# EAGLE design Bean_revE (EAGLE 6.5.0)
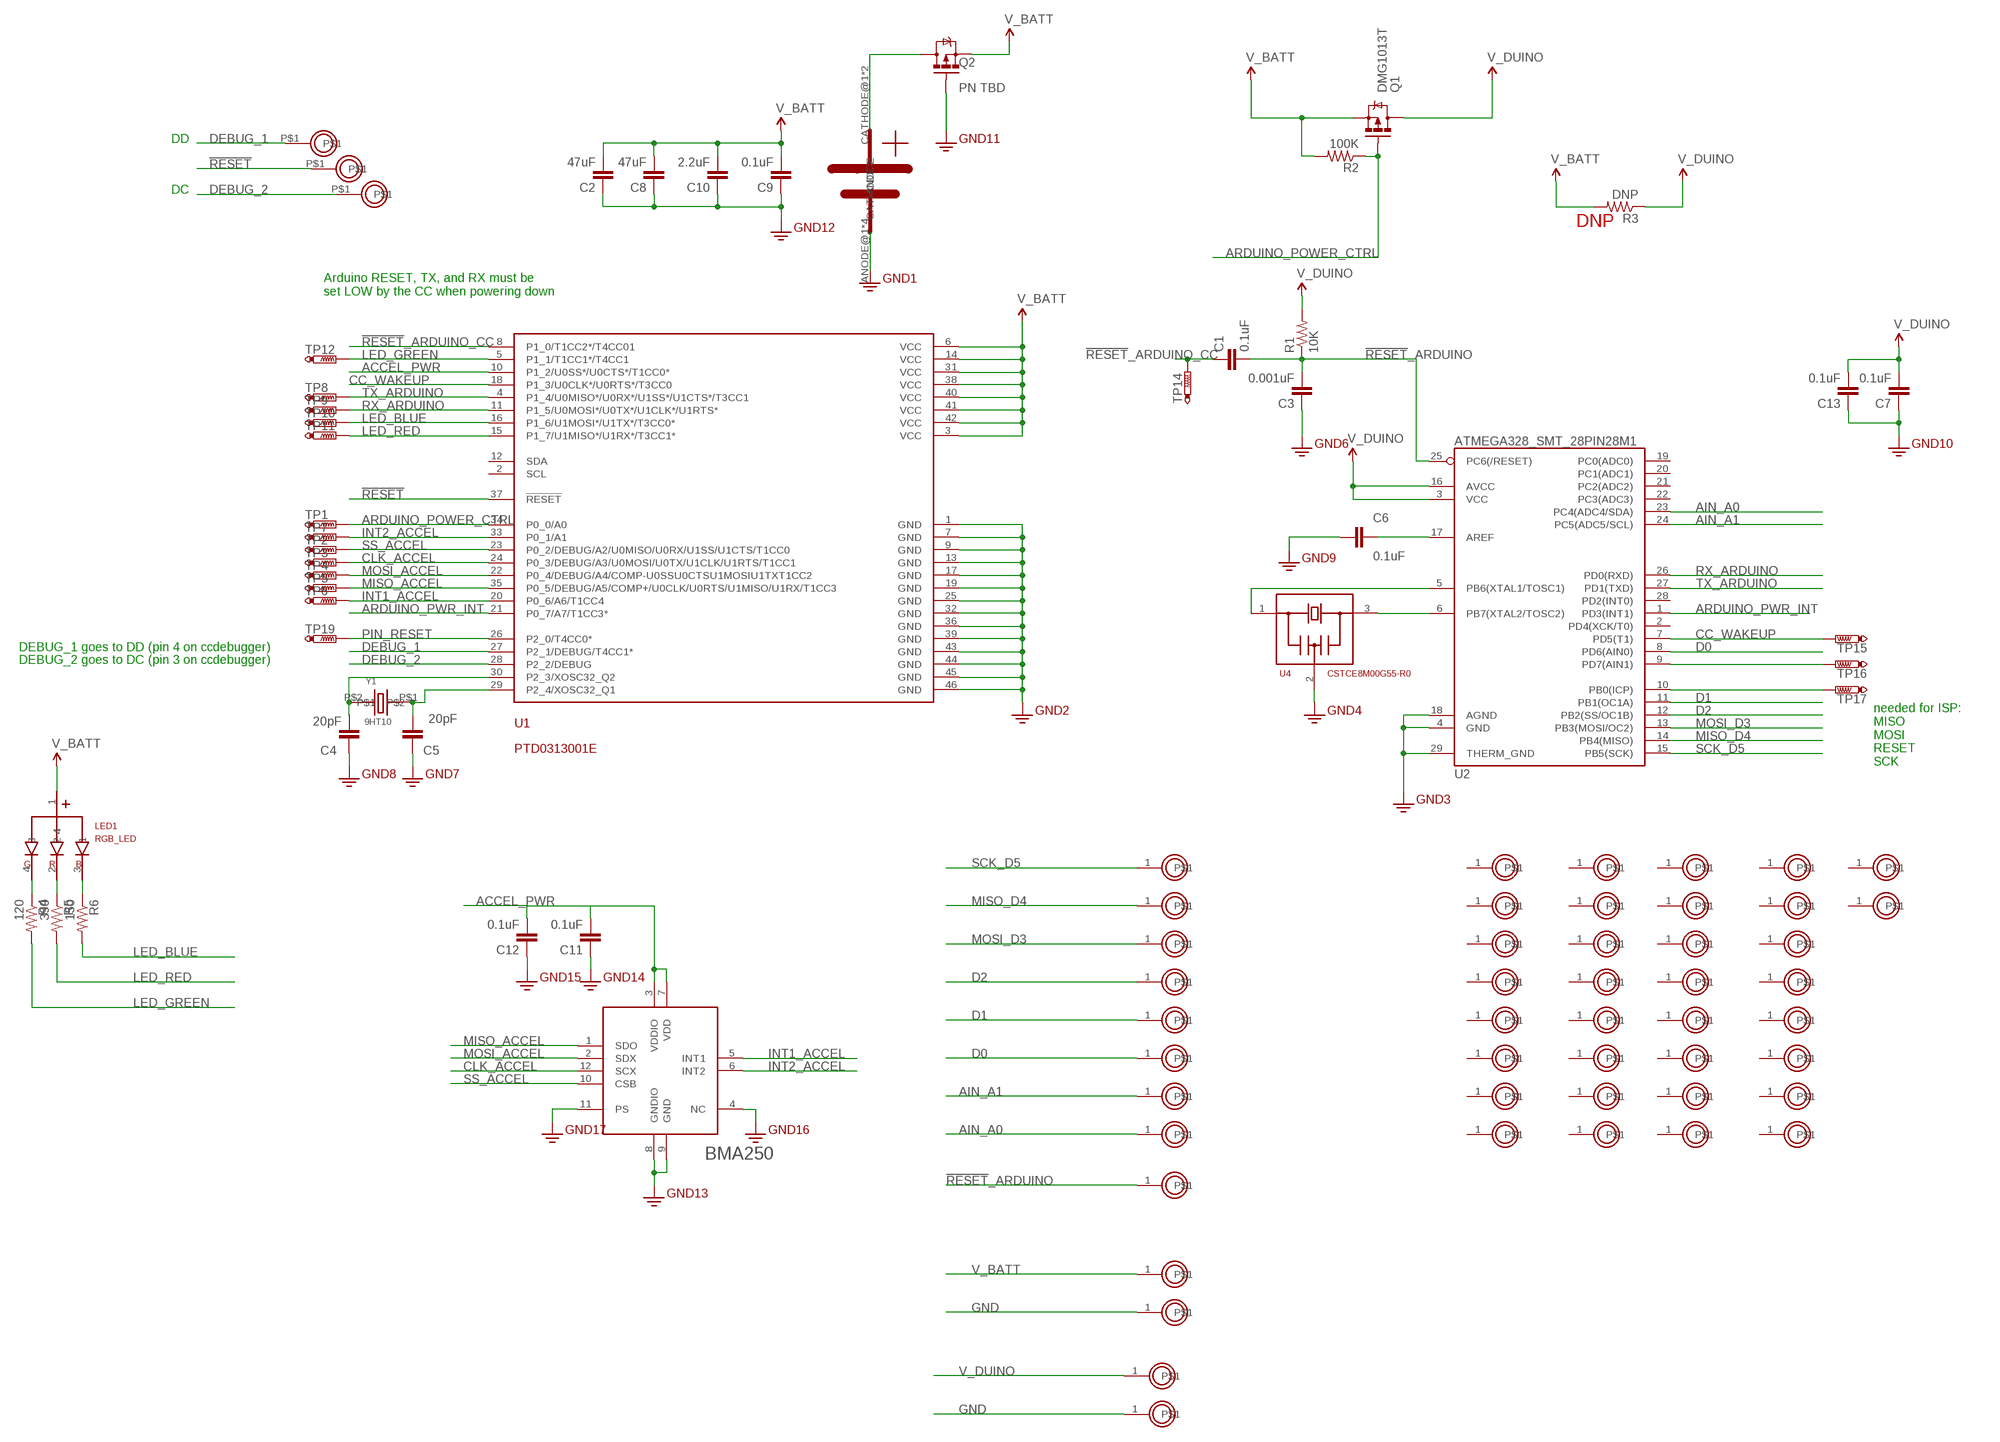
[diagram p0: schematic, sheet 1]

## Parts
C1  0.1uF  CAPACITOR_CERAMIC  [0402]
C2  47uF  CAP0805  [0805]
C3  0.001uF  CAPACITOR_CERAMIC  [0402]
C4  20pF  CAPACITOR_CERAMIC  [0402]
C5  20pF  CAPACITOR_CERAMIC  [0402]
C6  0.1uF  CAPACITOR_CERAMIC  [0402]
C7  0.1uF  CAPACITOR_CERAMIC  [0402]
C8  47uF  CAP0805  [0805]
C9  0.1uF  CAPACITOR_CERAMIC  [0402]
C10  2.2uF  CAP0603-CAP  [0603-CAP]
C11  0.1uF  CAPACITOR_CERAMIC  [0402]
C12  0.1uF  CAPACITOR_CERAMIC  [0402]
C13  0.1uF  CAPACITOR_CERAMIC  [0402]
CN_BATT  CR20324_ELEVATED_PADS  [BK-912-ALT]
LED1  RGB_LED  [SML-LX0404SIUPGUSB]
Q1  DMG1013T  MOSFET-PCHANNEL  [SOT523]
Q2  PN TBD  MOSFET-PCHANNEL  [SOT523]
R1  10K  RESISTOR  [0402]
R2  100K  RESISTOR  [0402]
R3  DNP  RESISTOR  [0402]
R4  120  RESISTOR  [0402]
R5  390  RESISTOR  [0402]
R6  150  RESISTOR  [0402]
TP1  PTR1TP06R  [TP06R]
TP2  PTR1TP06R  [TP06R]
TP3  PTR1TP06R  [TP06R]
TP4  PTR1TP06R  [TP06R]
TP5  PTR1TP06R  [TP06R]
TP6  PTR1TP06R  [TP06R]
TP7  PTR1TP06R  [TP06R]
TP8  PTR1TP06R  [TP06R]
TP9  PTR1TP06R  [TP06R]
TP10  PTR1TP06R  [TP06R]
TP11  PTR1TP06R  [TP06R]
TP12  PTR1TP06R  [TP06R]
TP14  PTR1TP06R  [TP06R]
TP15  PTR1TP06R  [TP06R]
TP16  PTR1TP06R  [TP06R]
TP17  PTR1TP06R  [TP06R]
TP19  PTR1TP14R  [TP14R]
U1  PTD0313001E  [PTD0313001E]
U2  ATMEGA328_SMT_28PIN28M1  [QFN-28-4X4]
U3  BMA250  [BMA250]
U4  CSTCE8M00G55-R0  RESONATOR_3PIN  [CSTCE_G_3PIN_XTAL]
U$1  PROTO_POINT  [1X01]
U$3  PROTO_POINT  [1X01]
U$4  PROTO_POINT  [1X01]
U$5  PROTO_POINT  [1X01]
U$6  PROTO_POINT  [1X01]
U$7  PROTO_POINT  [1X01]
U$8  PROTO_POINT  [1X01]
U$9  PROTO_POINT  [1X01]
U$10  PROTO_POINT  [1X01]
U$11  PROTO_POINT  [1X01]
U$12  PROTO_POINT  [1X01]
U$13  PROTO_POINT  [1X01]
U$14  PROTO_POINT  [1X01]
U$15  PROTO_POINT  [1X01]
U$16  PROTO_POINT  [1X01]
U$17  PROTO_POINT  [1X01]
U$18  PROTO_POINT  [1X01]
U$19  PROTO_POINT  [1X01]
U$20  PROTO_POINT  [1X01]
U$21  PROTO_POINT  [1X01]
U$22  PROTO_POINT  [1X01]
U$23  PROTO_POINT  [1X01]
U$24  PROTO_POINT  [1X01]
U$25  PROTO_POINT  [1X01]
U$26  PROTO_POINT  [1X01]
U$27  PROTO_POINT  [1X01]
U$28  PROTO_POINT  [1X01]
U$29  PROTO_POINT  [1X01]
U$30  PROTO_POINT  [1X01]
U$31  PROTO_POINT  [1X01]
U$32  PROTO_POINT  [1X01]
U$33  PROTO_POINT  [1X01]
U$34  PROTO_POINT  [1X01]
U$35  PROTO_POINT  [1X01]
U$36  PROTO_POINT  [1X01]
U$37  PROTO_POINT  [1X01]
U$38  PROTO_POINT  [1X01]
U$39  PROTO_POINT  [1X01]
U$40  PROTO_POINT  [1X01]
U$41  PROTO_POINT  [1X01]
U$42  PROTO_POINT  [1X01]
U$43  PROTO_POINT  [1X01]
U$44  PROTO_POINT  [1X01]
U$45  PROTO_POINT  [1X01]
U$46  PROTO_POINT  [1X01]
U$49  BEAN_PROGRAM_PIN  [BEAN_PROGAM_PIN]
U$50  BEAN_PROGRAM_PIN  [BEAN_PROGAM_PIN]
U$51  BEAN_PROGRAM_PIN  [BEAN_PROGAM_PIN]
U$52  PROTO_POINT  [1X01]
U$53  PROTO_POINT  [1X01]
Y1  9HT10  [9HT10]

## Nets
!RESET!: U1.37(!RESET!) U$50.P$1
!RESET!_ARDUINO: C1.P$2 C3.P$2 R1.P$1 U2.25(PC6(/RESET)) U$46.1
!RESET!_ARDUINO_CC: C1.P$1 TP14.TP U1.8(P1_0/T1CC2*/T4CC01)
ACCEL_PWR: C11.P$2 C12.P$2 U1.10(P1_2/U0SS*/U0CTS*/T1CC0*) U3.3(VDDIO) U3.7(VDD)
AIN_A0: U2.23(PC4(ADC4/SDA)) U$10.1
AIN_A1: U2.24(PC5(ADC5/SCL)) U$9.1
ARDUINO_POWER_CTRL: Q1.G R2.P$1 TP1.TP U1.34(P0_0/A0)
ARDUINO_PWR_INT: U1.21(P0_7/A7/T1CC3*) U2.1(PD3(INT1))
CC_WAKEUP: TP15.TP U1.18(P1_3/U0CLK*/U0RTS*/T3CC0) U2.7(PD5(T1))
CLK_ACCEL: TP3.TP U1.24(P0_3/DEBUG/A3/U0MOSI/U0TX/U1CLK/U1RTS/T1CC1) U3.12(SCX)
D0: U2.8(PD6(AIN0)) U$8.1
D1: U2.11(PB1(OC1A)) U$7.1
D2: U2.12(PB2(SS/OC1B)) U$6.1
DEBUG_1: U1.27(P2_1/DEBUG/T4CC1*) U$51.P$1
DEBUG_2: U1.28(P2_2/DEBUG) U$49.P$1
GND: C2.1 C3.P$1 C4.P$1 C5.P$1 C6.P$1 C7.P$1 C8.1 C9.P$1 C10.1 C11.P$1 C12.P$1 C13.P$1 CN_BATT.ANODE@1(ANODE) CN_BATT.ANODE@2(ANODE) CN_BATT.ANODE@3(ANODE) CN_BATT.ANODE@4(ANODE) Q2.G U1.1(GND) U1.7(GND) U1.9(GND) U1.13(GND) U1.17(GND) U1.19(GND) U1.25(GND) U1.32(GND) U1.36(GND) U1.39(GND) U1.43(GND) U1.44(GND) U1.45(GND) U1.46(GND) U2.4(GND) U2.18(AGND) U2.29(THERM_GND) U3.4(NC) U3.8(GNDIO) U3.9(GND) U3.11(PS) U4.2 U$45.1 U$53.1 ; supply symbol labelled GND2
INT1_ACCEL: TP6.TP U1.20(P0_6/A6/T1CC4) U3.5(INT1)
INT2_ACCEL: TP7.TP U1.33(P0_1/A1) U3.6(INT2)
LED_BLUE: R6.P$2 TP10.TP U1.16(P1_6/U1MOSI*/U1TX*/T3CC0*)
LED_GREEN: R4.P$2 TP12.TP U1.5(P1_1/T1CC1*/T4CC1)
LED_RED: R5.P$2 TP11.TP U1.15(P1_7/U1MISO*/U1RX*/T3CC1*)
MISO_ACCEL: TP5.TP U1.35(P0_5/DEBUG/A5/COMP+/U0CLK/U0RTS/U1MISO/U1RX/T1CC3) U3.1(SDO)
MISO_D4: U2.14(PB4(MISO)) U$4.1
MOSI_ACCEL: TP4.TP U1.22(P0_4/DEBUG/A4/COMP-U0SSU0CTSU1MOSIU1TXT1CC2) U3.2(SDX)
MOSI_D3: U2.13(PB3(MOSI/OC2)) U$5.1
N$1: U2.5(PB6(XTAL1/TOSC1)) U4.1
N$2: U2.6(PB7(XTAL2/TOSC2)) U4.3
N$3: C4.P$2 U1.30(P2_3/XOSC32_Q2) Y1.P$2
N$4: C5.P$2 U1.29(P2_4/XOSC32_Q1) Y1.P$1
N$6: C6.P$2 U2.17(AREF)
N$23: LED1.4 R4.P$1
N$24: LED1.2 R5.P$1
N$25: LED1.3 R6.P$1
PB0: TP17.TP U2.10(PB0(ICP))
PD7: TP16.TP U2.9(PD7(AIN1))
PIN_RESET: TP19.TP U1.26(P2_0/T4CC0*)
PRE_V_BATT: CN_BATT.CATHODE@1(CATHODE) CN_BATT.CATHODE@2(CATHODE) Q2.D
RX_ARDUINO: TP9.TP U1.11(P1_5/U0MOSI*/U0TX*/U1CLK*/U1RTS*) U2.26(PD0(RXD))
SCK_D5: U2.15(PB5(SCK)) U$3.1
SS_ACCEL: TP2.TP U1.23(P0_2/DEBUG/A2/U0MISO/U0RX/U1SS/U1CTS/T1CC0) U3.10(CSB)
TX_ARDUINO: TP8.TP U1.4(P1_4/U0MISO*/U0RX*/U1SS*/U1CTS*/T3CC1) U2.27(PD1(TXD))
V_BATT: C2.2 C8.2 C9.P$2 C10.2 LED1.1 Q1.S Q2.S R2.P$2 R3.P$2 U1.3(VCC) U1.6(VCC) U1.14(VCC) U1.31(VCC) U1.38(VCC) U1.40(VCC) U1.41(VCC) U1.42(VCC) U$52.1
V_DUINO: C7.P$2 C13.P$2 Q1.D R1.P$2 R3.P$1 U2.3(VCC) U2.16(AVCC) U$1.1
Unconnected: U1.2(SCL) U1.12(SDA) U2.2(PD4(XCK/T0)) U2.19(PC0(ADC0)) U2.20(PC1(ADC1)) U2.21(PC2(ADC2)) U2.22(PC3(ADC3)) U2.28(PD2(INT0)) U$11.1 U$12.1 U$13.1 U$14.1 U$15.1 U$16.1 U$17.1 U$18.1 U$19.1 U$20.1 U$21.1 U$22.1 U$23.1 U$24.1 U$25.1 U$26.1 U$27.1 U$28.1 U$29.1 U$30.1 U$31.1 U$32.1 U$33.1 U$34.1 U$35.1 U$36.1 U$37.1 U$38.1 U$39.1 U$40.1 U$41.1 U$42.1 U$43.1 U$44.1

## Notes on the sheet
- DD
- DC
- DNP
- Arduino RESET, TX, and RX must be
  set LOW by the CC when powering down
- DEBUG_1 goes to DD (pin 4 on ccdebugger)
- DEBUG_2 goes to DC (pin 3 on ccdebugger)
- needed for ISP: 
  MISO
  MOSI
  RESET
  SCK

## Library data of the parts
C1 C3-C7 C9 C11-C13 = BLEduino Bean:CAPACITOR_CERAMIC
C2 C8 = BLEduino Bean:CAP: Capacitor
C10 = SparkFun-Capacitors:CAP: Capacitor
CN_BATT = BLEduino Bean:CR2032
LED1 = BLEduino Bean:RGB_LED
Q1 Q2 = BLEduino Bean:MOSFET-PCHANNEL: Generic PMOSFET
R1-R6 = BLEduino Bean:RESISTOR
TP1-TP12 TP14-TP17 TP19 = testpad:PTR1: TEST PIN
U1 = BLEduino Bean:PTD0313001E
U2 = BLEduino Bean:ATMEGA328_SMT_28PIN
U3 = BLEduino Bean:BMA250: Digital Accelerometer
U4 = BLEduino Bean:RESONATOR_3PIN
U$1 U$3-U$46 U$52 U$53 = BLEduino Bean:PROTO_POINT
U$49-U$51 = BeanLibrary:BEAN_PROGRAM_PIN
Y1 = BLEduino Bean:9HT10

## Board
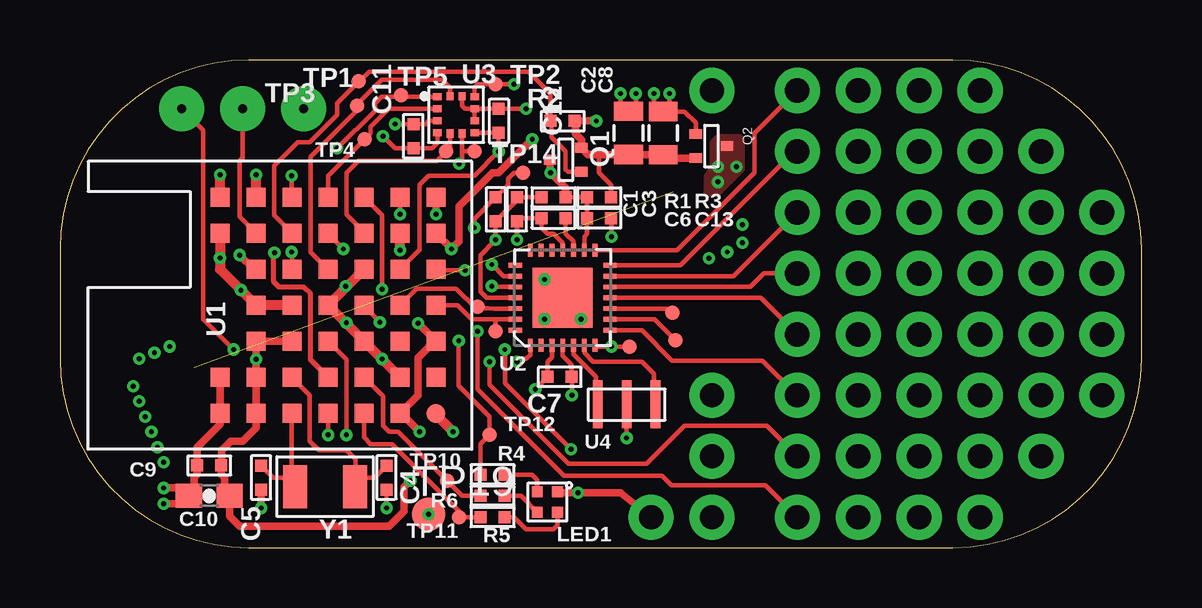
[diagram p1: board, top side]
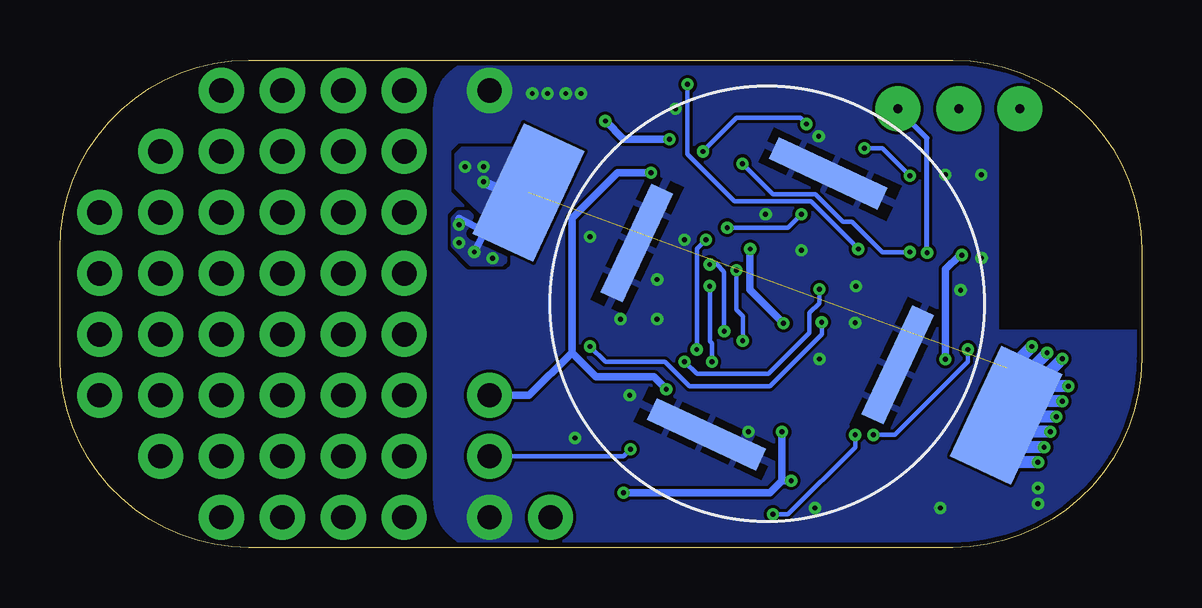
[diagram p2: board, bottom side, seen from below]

Size 45.09 x 20.32 mm. Coordinates in mm from the lower left corner, seen from the top.
Outline: 0,12.45 0,7.87 arc90 7.87,0 37.21,0 arc90 45.09,7.87 45.09,12.45 arc90 37.21,20.32 7.87,20.32 arc90 0,12.45
Copper layers (1*16): Top 0.035mm / dielectric 1.5mm / Bottom 0.035mm
Design rules "default *": minimum track width 7mil, minimum drill 0.15mm, track to track 5mil, track to pad 5mil, pad to pad 5mil, via to via 5mil, smd to smd 1mil, copper to edge 8mil, drill to drill 8mil, minimum pad ring 10mil, minimum via ring 2mil, stop-mask expansion 2mil, vias tented up to drill 13mil, thermal gap 10mil
tRestrict: area 1,10.7 to 5.6,15
bRestrict: area 1,10.7 to 5.6,15; area 8.3,8.7 to 9.4,10.1; area 9.2,9 to 10.3,10.5; area 8.9,7.3 to 10,8.7; area 9.8,7.6 to 10.9,9.1; area 9.5,5.9 to 10.7,7.3; area 10.4,6.2 to 11.5,7.7; area 10.2,4.5 to 11.3,5.9; area 11.1,4.9 to 12.2,6.3; area 19.1,13.9 to 20.2,15.3; area 20,14.2 to 21.1,15.7; area 19.7,12.5 to 20.8,13.9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

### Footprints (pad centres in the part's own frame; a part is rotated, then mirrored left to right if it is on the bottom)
0402 = smd 0.5 x 0.5: P$1 -0.5,0; P$2 0.5,0
0805 = smd 0.8 x 1.2: 1 -0.9,0; 2 0.9,0
0603-CAP = smd 1.1 x 1: 1 -0.85,0; 2 0.85,0
BK-912-ALT = smd 5 x 1: ANODE@1 0,6; ANODE@3 0,-6 | smd 1 x 5: ANODE@2 6,0; ANODE@4 -6,0 | smd 2.79 x 5.08: CATHODE@1 -10.985,0; CATHODE@2 10.985,0
SML-LX0404SIUPGUSB = smd 0.45 x 0.45: 1 0.425,0.425; 2 0.425,-0.425; 3 -0.425,-0.425; 4 -0.425,0.425
SOT523 = smd 0.4 x 0.51: D 0,0.65; G -0.5,-0.65; S 0.5,-0.65
TP06R = smd 0.6 x 0.6: TP 0,0
TP14R = smd 1.4 x 1.4: TP 0,0
PTD0313001E = smd 0.8 x 0.8: 1 1.5,1.5; 2 3,1.5; 3 4.5,1.5; 4 6,1.5; 5 7.5,1.5; 6 9,1.5; 7 10.5,1.5; 8 10.5,3; 9 9,3; 10 7.5,3; 11 6,3; 12 4.5,3; 13 3,3; 14 1.5,3; 15 1.5,4.5; 16 3,4.5; 17 4.5,4.5; 18 6,4.5; 19 7.5,4.5; 20 9,4.5; 21 10.5,4.5; 22 10.5,6; 23 9,6; 24 7.5,6; 25 6,6; 26 4.5,6; 27 3,6; 28 1.5,6; 29 1.5,7.5; 30 3,7.5; 31 4.5,7.5; 32 6,7.5; 33 7.5,7.5; 34 9,7.5; 35 10.5,7.5; 36 10.5,9; 37 9,9; 38 7.5,9; 39 6,9; 40 4.5,9; 41 3,9; 42 1.5,9; 43 1.5,10.5; 44 3,10.5; 45 9,10.5; 46 10.5,10.5
QFN-28-4X4 = smd 0.55 x 0.2: 1 -1.975,1.35; 2 -1.975,0.9; 3 -1.975,0.45; 4 -1.975,0; 5 -1.975,-0.45; 6 -1.975,-0.9; 7 -1.975,-1.35; 15 1.975,-1.35; 16 1.975,-0.9; 17 1.975,-0.45; 18 1.975,0; 19 1.975,0.45; 20 1.975,0.9; 21 1.975,1.35 | smd 0.2 x 0.55: 8 -1.35,-1.975; 9 -0.9,-1.975; 10 -0.45,-1.975; 11 0,-1.975; 12 0.45,-1.975; 13 0.9,-1.975; 14 1.35,-1.975; 22 1.35,1.975; 23 0.9,1.975; 24 0.45,1.975; 25 0,1.975; 26 -0.45,1.975; 27 -0.9,1.975; 28 -1.35,1.975 | smd 2.5 x 2.5: 29 0,0
BMA250 = smd 0.3 x 0.35: 1 -0.75,-0.775; 2 -0.25,-0.775; 3 0.25,-0.775; 4 0.75,-0.775; 7 0.75,0.775; 8 0.25,0.775; 9 -0.25,0.775; 10 -0.75,0.775 | smd 0.35 x 0.3: 5 0.775,-0.25; 6 0.775,0.25; 11 -0.775,0.25; 12 -0.775,-0.25
CSTCE_G_3PIN_XTAL = smd 0.4 x 2: 1 0.07,0; 2 1.27,0; 3 2.47,0
1X01 = drill 1.016 pad 1.88: 1 0,0
BEAN_PROGAM_PIN = drill 0.381 pad 1.88: P$1 0,0
9HT10 = smd 1 x 1.8: P$1 -1.25,0; P$2 1.25,0

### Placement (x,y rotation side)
C1  18.16,14.1 270 top
C2  23.7,17.28 270 top
C3  19.05,14.1 90 top
C4  13.61,2.92 90 top
C5  8.38,2.92 90 top
C6  20.57,13.72 0 top
C7  20.83,7.11 180 top
C8  25.15,17.27 270 top
C9  6.22,3.43 0 top
C10  6.22,2.16 0 top
C11  14.73,17.14 90 top
C12  18.29,17.78 270 top
C13  22.48,13.72 180 top
CN_BATT  15.6,10.16 335 bottom
LED1  20.32,1.91 0 top
Q1  21.08,16.16 90 top
Q2  27.15,16.73 270 top
R1  20.57,14.61 0 top
R2  20.95,17.78 0 top
R3  22.48,14.61 0 top
R4  18.03,3.05 180 top
R5  18.03,1.27 180 top
R6  18.03,2.16 180 top
TP1  12.45,19.43 0 top
TP2  18.16,19.3 0 top
TP3  12.38,18.41 0 top
TP4  12.7,17.02 0 top
TP5  14.22,18.85 0 top
TP6  16.1,16.51 0 top
TP7  17.27,16.51 0 top
TP8  18.16,9.02 0 top
TP9  17.4,10.03 0 top
TP10  16.13,2.79 0 top
TP11  16.64,1.27 0 top
TP12  17.91,4.7 0 top
TP14  19.3,15.62 0 top
TP15  23.75,8.38 0 top
TP16  25.65,8.64 0 top
TP17  25.53,9.78 0 top
TP19  15.37,1.4 0 top
U1  17.18,4.1 90 top
U2  20.95,10.41 90 top
U3  16.51,18.03 270 top
U4  22.35,5.97 0 top
U$1  27.18,6.35 0 top
U$3  30.73,19.05 0 top
U$4  30.73,16.51 0 top
U$5  30.73,13.97 0 top
U$6  30.73,11.43 0 top
U$7  30.73,8.89 0 top
U$8  30.73,6.35 0 top
U$9  30.73,3.81 0 top
U$10  30.73,1.27 0 top
U$11  33.27,19.05 0 top
U$12  35.81,19.05 0 top
U$13  33.27,11.43 0 top
U$14  33.27,16.51 0 top
U$15  35.81,16.51 0 top
U$16  35.81,11.43 0 top
U$17  33.27,13.97 0 top
U$18  35.81,13.97 0 top
U$19  33.27,1.27 90 top
U$20  33.27,3.81 90 top
U$21  33.27,6.35 90 top
U$22  33.27,8.89 90 top
U$23  38.35,13.97 0 top
U$24  35.81,1.27 90 top
U$25  35.81,3.81 90 top
U$26  35.81,6.35 90 top
U$27  35.81,8.89 90 top
U$28  38.35,16.51 0 top
U$29  38.35,11.43 90 top
U$30  38.35,3.81 90 top
U$31  38.35,6.35 90 top
U$32  38.35,8.89 90 top
U$33  40.89,16.51 0 top
U$34  40.89,13.97 0 top
U$35  40.89,6.35 0 top
U$36  40.89,11.43 0 top
U$37  40.89,3.81 0 top
U$38  40.89,8.89 0 top
U$39  38.35,19.05 0 top
U$40  43.43,13.97 0 top
U$41  38.35,1.27 0 top
U$42  43.43,11.43 0 top
U$43  43.43,8.89 0 top
U$44  43.43,6.35 0 top
U$45  27.18,19.05 0 top
U$46  27.18,3.81 0 top
U$49  5.08,18.29 0 top
U$50  7.62,18.29 0 top
U$51  10.16,18.29 0 top
U$52  24.64,1.27 0 top
U$53  27.18,1.27 0 top
Y1  11.05,2.54 0 top

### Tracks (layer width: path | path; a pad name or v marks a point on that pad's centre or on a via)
!RESET!
  Top 0.178: U1.37 7.49,13.78 7.49,16.13 7.62,16.26 U$50.P$1
  Top 0.203: U1.37 8.11,13.1
!RESET!_ARDUINO  (via drill 0.2 pad 0.51)
  Top 0.178: R1.P$1 19.18,14.61 C3.P$2 19.05,14.49 C1.P$2 v18.16,12.83 17.53,12.19 17.53,10.67 17.78,10.41 U2.25 | v18.54,8.27 v18.54,8.26 18.54,6.86 v21.3,4.1
  Bottom 0.178: v18.54,8.26 18.54,12.45 v18.16,12.83 | v21.3,4.1 21.59,3.81 U$46.1
!RESET!_ARDUINO_CC  (via drill 0.2 pad 0.51)
  Top 0.178: v17.27,13.34 17.27,13.71 C1.P$1 18.67,15.11 18.67,15.37 18.92,15.62 TP14.TP | U1.8 v14.18,13.9 v14.17,13.89
  Bottom 0.178: v17.27,13.34 14.73,13.34 v14.17,13.89
ACCEL_PWR  (via drill 0.2 pad 0.51)
  Top 0.178: U3.7 C12.P$2 v18.29,16.51 17.27,15.49 15.37,15.49 14.99,15.11 14.99,12.41 U1.10 | U3.3 15.37,17.78 15.23,17.64 C11.P$2 14.72,17.65 v13.97,17.65
  Bottom 0.178: v18.29,16.51 16.89,17.91 14.22,17.91 v13.97,17.65
AIN_A0  (via drill 0.2 pad 0.51)
  Top 0.178: v18,11.8 18.49,11.31 U2.23 | U$10.1 29.4,2.6 25.49,2.6 25.09,3 21,3 17.4,6.6 v17.4,9.02
  Bottom 0.178: v18,11.8 17.7,11.8 17.4,11.5 v17.4,9.02
AIN_A1  (via drill 0.2 pad 0.51)
  Top 0.178: v18,10.9 18.04,10.86 U2.24 | U$9.1 29.46,5.08 26.04,5.08 24.45,3.5 21.2,3.5 17.91,6.79 v17.91,7.75
  Bottom 0.178: v18,10.9 18,8.6 17.91,8.51 v17.91,7.75
ARDUINO_POWER_CTRL
  Top 0.178: U1.34 8.93,13.85 8.93,15.91 9.91,16.89 10.41,16.89 11.56,18.03 11.56,18.52 12.39,19.36 | 12.39,19.36 12.88,19.84 19.53,19.84 20.45,18.92 R2.P$1 20.5,17.74 20.5,17.09 21.08,16.51 21.08,15.75 21.17,15.66 Q1.G | TP1.TP 12.45,19.36 12.39,19.36
ARDUINO_PWR_INT  (via drill 0.2 pad 0.51)
  Top 0.178: v13.43,10.77 13.43,13.85 U1.21 | v19.05,7.75 19.18,7.87 19.43,7.87 19.61,8.05 U2.1
  Bottom 0.178: v19.05,7.75 18.54,7.24 15.56,7.24 13.84,8.96 13.84,9.78 13.43,10.19 v13.43,10.77
CC_WAKEUP  (via drill 0.2 pad 0.51)
  Top 0.178: U1.18 12.68,10.06 v13.34,9.4 | U2.7 22.36,8.38 v22.99,8.38 TP15.TP
  Bottom 0.178: v13.34,9.4 13.34,8.89 15.49,6.73 18.85,6.73 19.86,7.75 22.35,7.75 v22.99,8.38
CLK_ACCEL
  Top 0.178: 10.96,11.6 U1.24 11.16,11.6 10.44,12.32 10.44,16.28 12.38,18.22 TP3.TP 12.38,18.48 13.41,19.51 15.93,19.51 16.26,19.17 U3.12
D0
  Top 0.178: U$8.1 29.29,7.8 25.52,7.8 24.25,9.06 U2.8
D1
  Top 0.178: U$7.1 29.21,10.41 U2.11
D2
  Top 0.178: U$6.1 29.34,11.43 28.77,10.86 U2.12
DEBUG_1  (via drill 0.2 pad 0.51)
  Top 0.203: U1.27 10.44,7.84 10.44,10.59 10.17,10.86 9.13,10.86 8.91,11.07 8.91,12.27 v8.94,12.29
  Bottom 0.203: v8.94,12.29 8.94,17.07 U$51.P$1
DEBUG_2  (via drill 0.2 pad 0.51)
  Top 0.178: U1.28 v11.18,4.7 | U$49.P$1 5.97,17.4 5.97,9.53 v7.24,8.26
  Bottom 0.178: v11.18,4.7 10.29,4.7 7.24,7.75 v7.24,8.26
GND  (via drill 0.2 pad 0.51)
  Top 0.178: U2.4 20.95,8 21.33,7.63 C7.P$1 v21.34,6.35 | U3.4 15.73,16.88 15.5,16.64 C11.P$1 | U3.9 C12.P$1 v19.43,18.29 | U3.9 U3.8 | U3.9 16.89,18.29 16.76,18.42 U3.11 | v19.05,12.83 C3.P$1 19.17,13.72 C6.P$1 20.07,13.33 20.32,13.08 20.57,13.08 20.95,12.7 U2.18 | U4.2 v23.62,4.57 | Q2.G 26.5,17.7 26.04,18.16 C8.1 | v23.37,18.92 23.37,18.51 C2.1 24,18.48 v24,18.92 | v24.77,18.92 24.77,18.54 25.14,18.17 C8.1 | v25.4,18.92 25.4,18.43 C8.1 | v22.99,12.95 22.99,13.71 C13.P$1 | v20.19,11.18 20.19,10.41 U2.29 | C11.P$1 | C11.P$1 13.96,16.64 v13.46,17.14 | C4.P$1 v13.61,1.65
  Top 0.305: U1.19 12.62,11.6 v11.91,10.89 | U1.44 U1.43 6.68,5.15 5.71,4.19 C9.P$1 5.72,3.06 5.59,2.92 5.59,2.37 | 5.59,2.37 C10.1 | C10.1 5.33,2.16 | 5.59,2.37 5.12,2.37 5.08,2.41 | v4.32,2.49 5.04,2.49 C10.1 | v4.32,1.83 5.04,1.83 C10.1 | C5.P$1 v8.38,1.65 | v15.67,13.89 U1.7
  Top 0.406: U1.19 U1.25 U1.17 U1.13 | U1.32 U1.39 6.68,11.6 v6.68,12.07 | v16.38,4.83 15.68,5.53 U1.1 | U1.45 v6.68,12.07 | v6.68,12.07 v6.67,12.07 | U1.36 v8.18,15.54 | v14.17,12.39 U1.9 | U1.46 v6.68,15.54
  Bottom 0.305: v8.38,1.65 8.51,1.65
  other vias: 11.94,9.37 13.43,7.86 7.54,10.73 20.19,9.53 21.72,9.53
  pour Bottom (rank 3, no thermals): 7.87,20.32 27.43,20.32 arc-90 29.46,18.29 29.46,2.03 arc-90 27.43,0 7.87,0 arc-93 0,8.26 0,12.57 arc-91
INT1_ACCEL
  Top 0.178: U1.20 12.68,13.13 11.94,13.87 11.94,15.62 12.45,16.13 15.72,16.13 TP6.TP 16.26,16.51 16.26,16.66 U3.5
INT2_ACCEL  (via drill 0.2 pad 0.51)
  Top 0.178: v16.64,16 16.76,16.12 16.76,16.51 | 16.76,16.51 U3.6 | U1.33 9.68,12.29 v9.65,12.32 | TP7.TP 16.76,16.51
  Bottom 0.178: v16.64,16 15.37,14.73 13.59,14.73 12.45,13.59 12.06,13.59 10.79,12.32 v9.65,12.32
LED_BLUE
  Top 0.178: U1.16 13.46,6.31 13.46,5.08 13.72,4.83 14.1,4.83 TP10.TP 16.76,2.16 R6.P$2
LED_GREEN  (via drill 0.2 pad 0.51)
  Top 0.178: U1.5 15.72,11.56 v16.89,11.56 | v16.62,8.62 16.62,6.74 17.91,5.46 TP12.TP 17.53,4.33 R4.P$2
  Bottom 0.178: v16.89,11.56 16.89,9.91 16.62,9.64 v16.62,8.62
LED_RED
  Top 0.178: 16.89,1.27 R5.P$2 TP11.TP 16.64,1.52 13.84,4.32 12.95,4.32 12.68,4.6 U1.15
MISO_ACCEL  (via drill 0.2 pad 0.51)
  Top 0.178: 9.68,14.82 U1.35 9.65,14.62 v9.65,15.49 | U3.1 14.29,18.78 | TP5.TP 14.29,18.78 | 14.29,18.78 13.4,18.78 13.13,18.52 13.13,18.21 v11.56,16.64
  Bottom 0.178: v9.65,15.49 10.79,16.64 v11.56,16.64
MISO_D4
  Top 0.178: U$4.1 30.61,16.51 25.86,11.76 U2.14
MOSI_ACCEL
  Top 0.178: U3.2 13.7,18.28 12.95,17.54 12.95,17.27 TP4.TP 11.18,15.49 U1.22
MOSI_D3
  Top 0.178: U$5.1 28.08,11.31 U2.13
N$1
  Top 0.178: U2.5 21.41,8.06 22.35,7.11 22.35,6.86 22.35,6.73 22.35,6.04 U4.1
N$2
  Top 0.178: U2.6 21.86,8.12 22.23,7.75 24.26,7.75 24.77,7.24 24.77,6.03 U4.3
N$3
  Top 0.178: 9.93,7.07 9.93,6.83 10.41,6.35 10.41,4.45 10.79,4.06 11.94,4.06 12.32,3.68 12.32,2.56 Y1.P$2 | Y1.P$2 12.3,2.65 12.32,2.67 | C4.P$2 13.11,2.92 12.3,2.92 Y1.P$2
  Top 0.254: U1.30 9.93,7.07
N$4
  Top 0.178: U1.29 9.65,5.58 9.65,3.05 9.8,2.9 Y1.P$1 | Y1.P$1 9.8,2.56 9.91,2.67 | C5.P$2 8.88,2.92 9.8,2.92 Y1.P$1
N$6
  Top 0.178: U2.17 21.41,12.76 21.08,13.08 21.08,13.71 C6.P$2
N$23
  Top 0.178: R4.P$1 19.68,3.05 19.89,2.84 LED1.4
N$24
  Top 0.178: R5.P$1 18.92,1.27 19.43,0.76 20.57,0.76 20.75,0.93 LED1.2
N$25
  Top 0.178: R6.P$1 19.22,2.16 LED1.3
PB0
  Top 0.178: U2.10 25.34,9.96 TP17.TP
PD7
  Top 0.178: U2.9 24.78,9.51 TP16.TP
PIN_RESET  (via drill 0.2 pad 0.51)
  Top 0.178: U1.26 11.94,7.84 v11.94,4.7 | 14.99,1.4 TP19.TP
  Bottom 0.178: v11.94,4.7 11.94,4.19 14.73,1.4 TP19.TP
  other vias: 15.37,1.4
PRE_V_BATT  (via drill 0.2 pad 0.51)  (1 unrouted)
  Bottom 0.305: CN_BATT.CATHODE@1 27.43,13.08 v27.81,12.32 27.3,13.34 27.43,13.21 28.45,13.72
  Bottom 0.406: 4.32,6.6 4.57,6.6 | 4.57,6.6 4.57,6.1 4.57,5.46 | 5.08,4.83 4.7,4.83 4.7,5.46 | 5.08,4.83 5.64,4.83 CN_BATT.CATHODE@2 | 5.08,4.83 5.08,4.32 | 5.08,4.19 5.21,4.19 5.21,3.56 | 5.59,7.49 5.08,7.49 5.08,6.99 5.08,6.6 4.57,6.6 | v27.43,15.24 26.29,14.73 | 26.29,14.73 arc-59 CN_BATT.CATHODE@1 | 26.29,14.73 arc62 26.16,13.59 26.23,13.45 arc-173 27.05,13.84
  Bottom 0.508: v3.05,6.73 4.32,6.73 | 4.32,6.73 4.32,6.6 | v3.3,6.1 4.57,6.1 | v3.56,5.46 4.57,5.46 4.7,5.46 | v3.81,4.83 5.08,4.83 | v4.06,4.19 5.08,4.19 5.08,4.32 | v4.32,3.56 5.21,3.56 5.33,3.56 5.33,3.43 | v3.3,7.87 4.32,6.86 4.32,6.73 | v3.94,8.13 5.08,6.99 5.21,6.86 | v4.57,8.38 5.46,7.49 5.59,7.49
  other vias: 27.43,15.88 28.19,15.88 28.45,12.7 27.05,12.06 28.45,13.46
  pour Top (no thermals): 28.32,17.14 27.43,17.14 27.18,16.89 27.18,15.88 26.92,15.49 26.92,14.73 27.43,14.73 28.45,15.75 28.45,17.02
  pour Bottom (no thermals): 26.42,15.37 26.67,14.61 26.8,14.35
  pour Bottom: 26.67,11.81 27.94,11.81 28.7,12.57 28.7,13.72 28.45,13.97 28.07,13.97 26.54,12.45 26.54,11.94
  pour Bottom (no thermals): 26.04,16.64 28.32,16.64 28.57,16.38 28.57,14.99 27.94,14.35 27.56,13.97 26.16,13.97 26.04,14.1
RX_ARDUINO
  Top 0.178: U2.26 18.09,9.96 17.84,9.97 17.4,9.97 | 17.4,9.97 17.34,9.97 16.51,10.79 14.87,10.79 U1.11 | TP9.TP 17.4,9.97
SCK_D5
  Top 0.178: U$3.1 28.96,17.27 28.96,15.62 25.72,12.39 U2.15
SS_ACCEL  (via drill 0.2 pad 0.51)
  Top 0.178: 11.18,13.07 U1.23 11.81,12.46 v11.81,12.45 | U3.10 17.29,19.19 17.4,19.3 TP2.TP v18.92,19.3
  Bottom 0.178: v11.81,12.45 13.79,14.43 16.97,14.43 18.92,16.38 v18.92,19.3
TX_ARDUINO
  Top 0.178: U2.27 18.16,9.51 | 18.16,9.51 17.16,9.51 16.57,10.1 U1.4 | TP8.TP 18.16,9.51
V_BATT  (via drill 0.2 pad 0.51)
  Top 0.178: 20.79,2.29 LED1.1 | R3.P$2 22.98,15.12 22.48,15.62 22.48,16.38
  Top 0.305: v14.92,9.35 U1.3 15.61,8.6 14.92,7.91 14.92,6.35 U1.14 14.21,5.6 v14.99,4.83 | Q2.S 25.29,16.23 C8.2 C2.2 22.48,16.38 22.01,16.38 Q1.S 21.73,17 21.5,17.24 21.5,17.74 R2.P$2 v22.35,17.78 | U1.31 U1.40 v8.18,7.85 U1.41 U1.42 8.18,5 7.62,4.45 7.11,4.45 6.73,4.06 C9.P$2 6.72,3.06 6.86,2.92 6.86,2.37 C10.2 7.07,1.31 7.49,0.89 13.72,0.89 14.35,1.52 14.35,2.54 v14.61,2.79 | v7.49,12.19 8.09,11.6 U1.38 | 20.79,2.29 v21.59,2.29 23.37,2.29 U$52.1 | v19.68,17.02 18.29,15.62 18.03,15.62 16.64,14.22 16.64,12.77 v16.32,12.45 15.68,13.09
  Top 0.406: 15.68,13.09 U1.6
  Bottom 0.305: v14.61,2.79 14.99,2.79 | 14.99,2.79 v14.99,4.83 | v8.18,7.85 U1.38 7.58,12.19 v7.49,12.19 | v19.68,17.02 21.59,17.02 v22.35,17.78 | v21.59,2.29 15.49,2.29 14.99,2.79 | v14.92,9.35 16.32,10.75 v16.32,12.45
V_DUINO  (via drill 0.2 pad 0.51)
  Top 0.178: U2.16 21.86,12.96 21.97,13.08 21.97,13.71 C13.P$2 R3.P$1 R1.P$2 | U2.3 20.5,7.93 20.32,7.75 C7.P$2 | C7.P$2 | C7.P$2 20.31,7.11 20.07,6.86 v19.81,6.6 | 20.43,15.64 20.43,15.62 v20.45,15.62
  Top 0.305: R1.P$2 21.07,14.99 v20.45,15.62 20.43,15.64 Q1.D
  Bottom 0.305: 23.75,8.13 23.75,13.72 21.84,15.62 v20.45,15.62 | U$1.1 25.53,6.35 23.75,8.13 | 23.75,8.13 22.73,7.11 C7.P$2 v19.81,6.6

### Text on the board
Document: Bean Revision E | ray@ | P/N: PTD1013012E | punchthrough.com | ck@ | Rev E | Top Silk: tPlace tArt | Bottom Silk: bArt | Layers: 2 | Rectangular Dimensions: 1.775" x 0.8" (45.09mm x 20.32mm) | Finished Thickness: 0.062" | Finish: ENIG | Material: FR4 | Copper Weight: 1oz | Soldermask: Top and bottom | Silkscreen: Top and Bottom | Silkscreen Color: Black | Soldermask Color: 85% white 10% green 5% blue | Min Drill: 0.008" | Min Annular Ring: 0.006" | Min Trace: 0.007" | Min Spacing: 0.005" | Corner mill radius: 0.32" | Avoid placing copper in antenna keepout
bArt: G / N / D | 5 | 4 | 3 | Rev E | 2 | VCC | 1 | 0 | R | A1 | BAT | G / N / D | A0
tArt: G / N / D | 5 | 4 | 3 | 2 | 1 | VCC | 0 | R | A1 | * | G / N / D | BAT | A0

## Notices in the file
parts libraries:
SparkFun-Aesthetics: Licensing: CC v3.0 Share-Alike You are welcome to use this library for commercial purposes.
